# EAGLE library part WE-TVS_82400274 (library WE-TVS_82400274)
TVS Diode Array WE-TVS, High Speed Series - Low capazity - No leakage current - Low clamping voltage - high ESD voltage protection -- USB 1.0 - 2.0 Double Port -- Ethernet
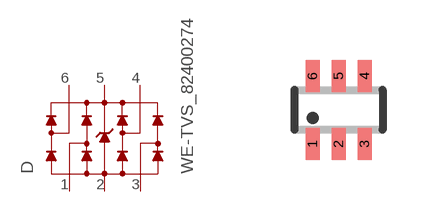
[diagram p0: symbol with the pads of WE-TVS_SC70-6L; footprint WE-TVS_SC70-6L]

Designator prefix D

## WE-TVS_82400274 (MPN: 82400274; OC_FARNELL: 1825876; OC_NEWARK: 79R6948; PACKAGE: SC70-6L; SUPPLIER: Wuerth Elektronik)  [WE-TVS_SC70-6L]
1  1  pas
2  GND  pwr
3  2  pas
4  3  pas
5  VDD  pwr
6  4  pas

## Footprint WE-TVS_SC70-6L (pad centres in mm)
TVS Diode Array WE-TVS
smd 0.35 x 0.8: 1 -0.65,-0.85; 2 0,-0.85; 3 0.65,-0.85; 4 0.65,0.85; 5 0,0.85; 6 -0.65,0.85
